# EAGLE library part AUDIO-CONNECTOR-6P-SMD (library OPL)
When you use the footprint ,place notice 46 (layer)milling ,there is some important information.
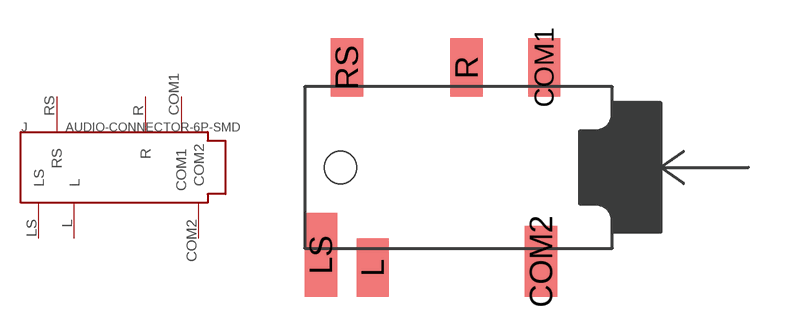
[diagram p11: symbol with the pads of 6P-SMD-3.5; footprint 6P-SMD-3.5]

Designator prefix J

## AUDIO-CONNECTOR-6P-SMD-3440030P1  [6P-SMD-3.5]
COM1  COM1
COM2  COM2
L  L
LS  LS
R  R
RS  RS

## Footprint 6P-SMD-3.5 (pad centres in mm)
smd 1.27 x 2.286: COM1 2.413,3.937; L -4.318,-3.937; R -0.635,3.937; RS -5.334,3.937
smd 1.27 x 2.794: COM2 2.286,-3.683
smd 1.27 x 3.302: LS -6.35,-3.429
hole 1.27 at -5.588,0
